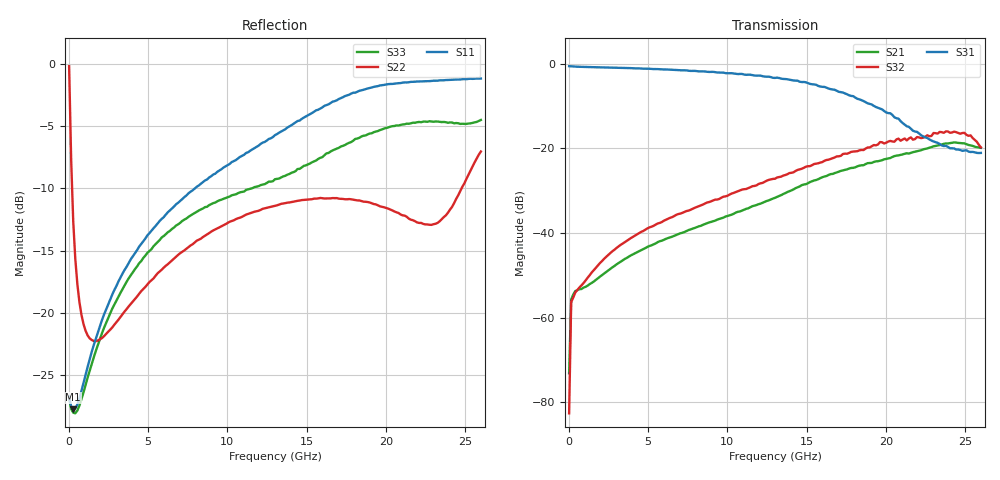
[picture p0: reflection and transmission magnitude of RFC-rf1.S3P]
!  3-Port S-parameters saved by WinCal
! VAR MeasName=S-Parameters (CALIBRATED_DATA) read from VNA (N5245A)
! VAR MeasDate=2016-7-4 10:41:01
! VAR NAME=25_C168105_RF1_RF4_00
! VAR FILENAME=25_C168105_RF1_RF4_00.S3P
! VAR DATE=2016-7-4 10:41:01
! VAR PHYS_PORTS=1,2,3
# Hz S DB R 50
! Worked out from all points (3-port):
!   201 points, 10 MHz to 26 GHz, reference 50 ohm
!   strongest paths, dB at 10 MHz, 6.508 GHz, 13.01 GHz, 19.5 GHz, 26 GHz:
!     S31: -0.6, -1.4, -3.3, -10.4, -21.1
!     S32: -82.6, -36.3, -27.2, -19.1, -19.8
!     S21: -73.1, -40.9, -31.7, -23.0, -19.9
!   lowest |S11| = -27.8 dB at 269.9 MHz (marker M1), VSWR 1.09, Z = 53.5 - j2.34 ohm
!   |S11| at or under -10 dB: start of sweep to 7.952 GHz
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1e7  -26.75 -5.0  -75.69 85.4  -0.57 -0.3
     -73.15 72.6  -0.19 -9.2  -85.62 91.3
     -0.57 -0.3  -82.61 60.3  -26.87 -4.2
1.3995e8  -27.55 -19.0  -55.65 41.4  -0.61 -2.0
          -55.73 41.8  -7.75 -65.6  -56.36 45.5
          -0.61 -2.0  -56.31 44.6  -27.73 -17.6
2.699e8  -27.76 -32.1  -54.86 29.6  -0.65 -3.6
         -54.55 30.0  -12.67 -77.2  -55.01 36.0
         -0.65 -3.7  -55.26 36.4  -28.03 -29.7
7.897e8  -26.28 -64.0  -53.12 27.5  -0.74 -9.5
         -53.23 27.6  -20.17 -88.0  -52.37 41.2
         -0.73 -9.6  -52.38 41.7  -26.92 -59.4
1.5694e9  -22.58 -88.6  -51.45 39.7  -0.81 -18.3
          -51.46 39.8  -22.27 -94.5  -48.74 51.8
          -0.81 -18.4  -48.79 51.9  -23.57 -83.7
6.7674e9  -11.28 -162.5  -40.49 43.0  -1.48 -77.2
          -40.46 43.3  -15.49 -133.1  -35.70 25.4
          -1.45 -76.9  -35.71 25.6  -12.99 -160.5
1.3005e10  -5.73 138.2  -31.90 18.9  -3.43 -150.0
           -31.68 18.0  -11.40 173.5  -27.15 -35.1
           -3.35 -150.7  -27.18 -34.5  -9.27 94.0
1.807305e10  -2.32 90.8  -24.83 -29.6  -8.68 142.5
             -24.47 -28.0  -10.95 117.1  -21.06 -100.8
             -8.00 143.3  -20.70 -101.1  -6.03 -20.6
2.13218e10  -1.50 60.0  -21.18 -58.3  -14.77 122.9
            -21.15 -62.5  -12.29 77.4  -17.98 -154.1
            -14.77 116.5  -18.12 -156.1  -4.81 -79.0
2.6e10  -1.18 22.4  -19.90 -112.5  -20.92 154.8
        -19.87 -115.5  -7.05 39.2  -19.61 94.2
        -21.07 150.2  -19.76 93.5  -4.51 -130.2
